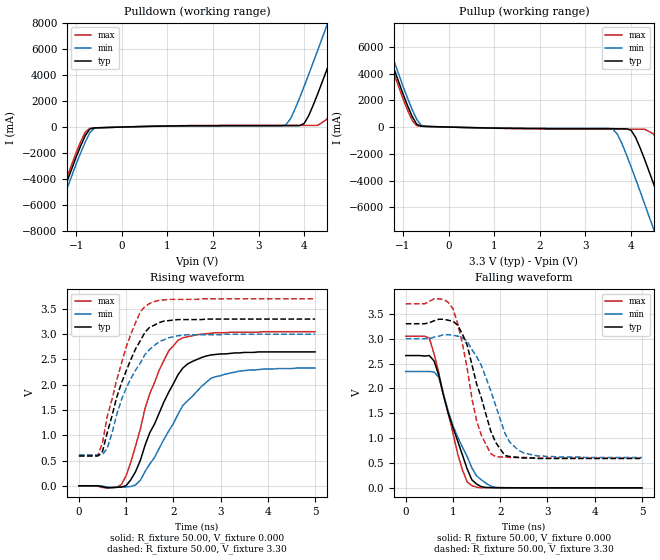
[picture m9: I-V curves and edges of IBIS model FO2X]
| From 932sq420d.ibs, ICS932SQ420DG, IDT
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|   Model FO2X
[Model]   FO2X
Model_type   Output
Polarity   Non-Inverting
Vmeas =   1.50V
C_comp   3.40pF   2.85pF   3.95pF
[Temperature Range]   27.00   70.00   0.000
[Voltage Range]   3.30V   3.00V   3.70V
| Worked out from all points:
|   slope of the pulldown table from 0 to 0.495 V, typ, clamps not added: 10.5 ohm
|   slope of the pullup table from 0 to 0.495 V, typ, clamps not added: 11.7 ohm
|   rising waveform, R_fixture 50.00, V_fixture 0.000: 20-80 % time 746ps typ, 966ps min, 635ps max; typ from 0 V to 2.65 V
|   rising waveform, R_fixture 50.00, V_fixture 3.30: 20-80 % time 605ps typ, 641ps min, 564ps max; typ from 0.59 V to 3.3 V
|   falling waveform, R_fixture 50.00, V_fixture 0.000: 20-80 % time 514ps typ, 568ps min, 456ps max; typ from 2.66 V to 0 V
|   falling waveform, R_fixture 50.00, V_fixture 3.30: 20-80 % time 475ps typ, 541ps min, 390ps max; typ from 3.3 V to 0.59 V
[Pulldown]
| voltage   I(typ)   I(min)   I(max)
-3.3V     -24.68A    -25.2A     -24.36A
-1.7V     -8.95A     -9.49A     -8.61A
-1.5V     -7.01A     -7.56A     -6.67A
-900mV    -1.43A     -1.97A     -1.11A
-700mV    -150mA     -440mA     -91.09mA
3.6V      110mA      170mA      130mA
4V        270mA      3.13A      130mA
4.3V      2.57A      5.93A      130mA
4.5V      4.43A      7.85A      600mA
4.9V      8.27A      11.73A     4.09A
5.3V      12.17A     15.65A     7.94A
6.6V      25.02A     28.51A     20.75A
[Pullup]
| voltage   I(typ)   I(min)   I(max)
-3.3V     24.86A     25.41A     24.53A
-1.7V     9.13A      9.7A       8.77A
-1.5V     7.19A      7.77A      6.83A
-900mV    1.59A      2.15A      1.25A
-700mV    210mA      570mA      100mA
3.6V      -120mA     -150mA     -160mA
4V        -230mA     -2.95A     -160mA
4.3V      -2.42A     -5.75A     -160mA
4.5V      -4.27A     -7.66A     -520mA
4.9V      -8.1A      -11.54A    -3.96A
5.3V      -12A       -15.45A    -7.8A
6.6V      -24.81A    -28.28A    -20.57A
[Ramp]
| variable   typ   min   max
dV/dt_r   1.59/0.75n   1.40/0.95n   1.83/0.63n
dV/dt_f   1.63/0.46n   1.43/0.55n   1.86/0.40n
R_load = 50.00
[Rising Waveform]
R_fixture = 50.00
V_fixture = 0.000
V_fixture_min = 0.000
V_fixture_max = 0.000
| time   V(typ)   V(min)   V(max)
0s        0V         0V         0V
900ps     -24.61mV   -25.36mV   24.72mV
1.2ns     280mV      17.23mV    790mV
1.5ns     1.05V      430mV      1.82V
1.9ns     1.85V      1.08V      2.67V
2.1ns     2.2V       1.42V      2.88V
2.3ns     2.41V      1.68V      2.95V
2.8ns     2.59V      2.13V      3.02V
3.6ns     2.64V      2.29V      3.04V
5ns       2.65V      2.33V      3.05V
[Rising Waveform]
R_fixture = 50.00
V_fixture = 3.30
V_fixture_min = 3.00
V_fixture_max = 3.70
| time   V(typ)   V(min)   V(max)
0s        590mV      610mV      600mV
400ps     590mV      610mV      600mV
500ps     680mV      620mV      850mV
600ps     1.05V      740mV      1.37V
1ns       2.27V      1.93V      2.74V
1.3ns     2.87V      2.43V      3.44V
1.4ns     3.04V      2.6V       3.55V
1.7ns     3.23V      2.85V      3.67V
2.1ns     3.29V      2.97V      3.69V
5ns       3.3V       3V         3.7V
[Falling Waveform]
R_fixture = 50.00
V_fixture = 0.000
V_fixture_min = 0.000
V_fixture_max = 0.000
| time   V(typ)   V(min)   V(max)
0s        2.66V      2.34V      3.05V
500ps     2.66V      2.34V      3.01V
600ps     2.55V      2.33V      2.69V
700ps     2.26V      2.22V      2.31V
900ps     1.5V       1.54V      1.49V
1.1ns     940mV      1.02V      680mV
1.3ns     380mV      630mV      120mV
1.4ns     160mV      400mV      43.44mV
1.9ns     3.32mV     6.5mV      2.61mV
5ns       -3.61uV    6.69uV     -5.25uV
[Falling Waveform]
R_fixture = 50.00
V_fixture = 3.30
V_fixture_min = 3.00
V_fixture_max = 3.70
| time   V(typ)   V(min)   V(max)
0s        3.3V       3V         3.7V
700ps     3.39V      3.05V      3.8V
1ns       3.35V      3.07V      3.6V
1.3ns     2.87V      2.95V      2.4V
1.5ns     2.09V      2.64V      1.35V
1.8ns     1.14V      1.95V      690mV
2.1ns     650mV      1.1V       620mV
2.2ns     630mV      920mV      610mV
2.5ns     600mV      700mV      610mV
5ns       590mV      610mV      600mV
